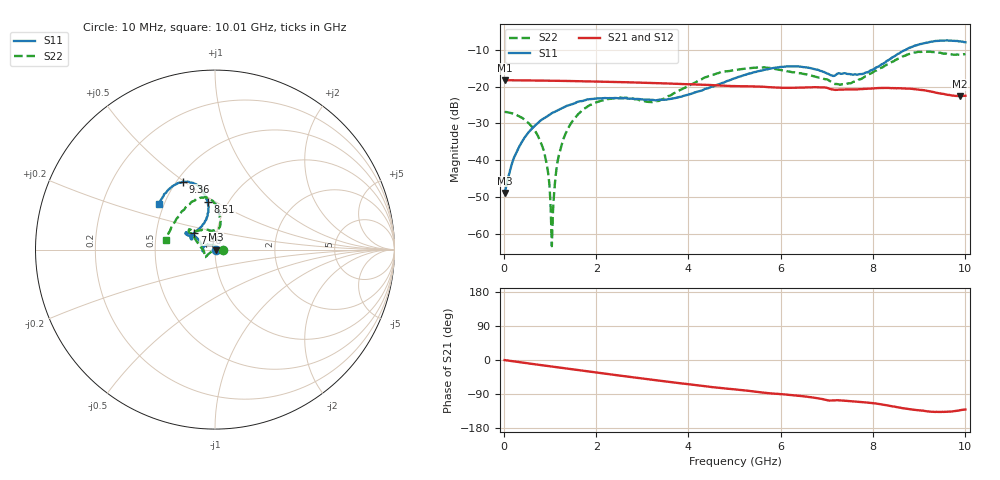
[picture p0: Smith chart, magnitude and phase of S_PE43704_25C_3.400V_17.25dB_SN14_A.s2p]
! Device ID: PE43704
! Dir: z:\PE43704\PE43704_Char_1_20130516\PE43704\AMB\3p400V\17p25dB
! Serial: 14
! Insertion: A
! Impedance: 50 ohm
! Temp: Amb
! VDD: 3.400V
! Attenuation Step: 17.25dB
! IDD: 1.139146e-01mA
#  Hz  S  RI  R  50
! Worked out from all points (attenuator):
!   401 points, 10 MHz to 10.01 GHz, reference 50 ohm
!   highest |S21| = -18.23 dB at 10 MHz (marker M1); lowest = -22.6 dB at 9.885 GHz (marker M2)
!   lowest |S11| = -48.9 dB at 10 MHz (marker M3), VSWR 1.01, Z = 50.4 + j0.0479 ohm
!   |S11| at or under -10 dB: start of sweep to 8.714 GHz
!   |S22| runs from -63.4 to -10.4 dB; largest |S21 - S12| = 0.0013
!   S11 on the Smith chart (normalised r, x): 10 MHz: 1.01, +0.00; 7.46 GHz: 0.78, +0.15; 8.51 GHz: 0.81, +0.46; 9.36 GHz: 0.54, +0.49; 10.01 GHz: 0.47, +0.28
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1e7  0.00356 0.000475  0.1226 -0.00042  0.1226 -0.000317  0.0453 -3.44e-05
2.85e8  0.000906 0.0134  0.1215 -0.0104  0.1215 -0.0104  0.0405 0.00439
7.35e8  -0.0153 0.0283  0.1182 -0.0261  0.1182 -0.026  0.0206 0.00566
9.1e8  -0.0247 0.0297  0.1164 -0.0319  0.1164 -0.0318  0.00931 0.00273
9.6e8  -0.0272 0.0301  0.1159 -0.0334  0.1159 -0.0334  0.0062 0.00148
9.85e8  -0.0287 0.0303  0.1156 -0.0343  0.1156 -0.0343  0.00432 0.00117
1.035e9  -0.0319 0.0298  0.1151 -0.0359  0.115 -0.0358  0.000319 -0.000599
1.085e9  -0.0344 0.0293  0.1144 -0.0376  0.1144 -0.0375  -0.00286 -0.00226
1.16e9  -0.0384 0.0285  0.1133 -0.04  0.1133 -0.0399  -0.00838 -0.00484
1.26e9  -0.0435 0.0269  0.1118 -0.0433  0.1118 -0.0432  -0.0151 -0.00817
1.685e9  -0.0619 0.0151  0.1046 -0.0557  0.1046 -0.0557  -0.0391 -0.0268
2.36e9  -0.0698 -0.00389  0.0904 -0.0727  0.0905 -0.0727  -0.0555 -0.0417
3.36e9  -0.0664 -0.000861  0.0648 -0.0906  0.0648 -0.0906  -0.0639 -0.00619
5.01e9  -0.1087 0.0717  0.0218 -0.0993  0.022 -0.0995  -0.1411 0.0925
5.96e9  -0.1566 0.0956  0.000763 -0.0967  0.000896 -0.097  -0.1328 0.1063
6.685e9  -0.1569 0.0824  -0.0151 -0.097  -0.0149 -0.0968  -0.0928 0.1054
7.46e9  -0.1149 0.0943  -0.0287 -0.0871  -0.0285 -0.0872  0.00339 0.1106
8.36e9  -0.0366 0.2308  -0.0491 -0.0824  -0.0492 -0.0827  0.0221 0.2063
8.51e9  -0.0394 0.266  -0.0534 -0.0786  -0.0533 -0.0796  0.0122 0.2331
9.36e9  -0.1785 0.378  -0.0608 -0.0567  -0.0611 -0.0568  -0.1335 0.2635
9.885e9  -0.2923 0.2915  -0.0504 -0.0547  -0.0509 -0.0545  -0.2499 0.1068
1.001e10  -0.3116 0.2529  -0.0488 -0.0573  -0.0495 -0.0574  -0.2717 0.0561
